ORGANIZATION_BLOCK MAIN:OB1
TITLE= Ciclo elettropneumatico A+/B+/A-/B- (ciclo quadro)
// Simulatore: 05
// Versione: 1.0
// Data: 28/02/2002
//------------     DESCRIZIONE  ---------------------
// L'esempio utilizza due cilindri (A e B) a doppio effetto e due
// elettrovalvole 5/2 bistabili (1V1 e 2V1).
// Una valvola 3/2 monostabile 0V permette la distribuzione dell'aria al
// circuito.
// Sulla mandata di ciascun cilindro sono preseti degli strozzatori
// unidirezionali che permettono di regolare separatamente la velocità
// delle singole corse dei pistoni.
// Un circuito di sicurezza, esterno al PLC, provvede (quando disattivato)
// a far rientrare lo stelo dei cilindri nella posizione di riposo
// (A0 B0)indipendentemente dalle uscite del PLC che vengono invece
// disattivate mediante un contatto del circuito di sicurezza
// (simulato dal Pulsante SB5). L'intervento di detto circuito
// non toglie però l'erogazione dell'aria compressa al circuito.
// Il ciclo continuo inizia con la pressione del pulsante SB1 e potrà
// essere interrotto mediante il pulsante di Stop SB3.
// Il pulsante SB2 permette di effetuare un solo ciclo quando premuto.
// Agli ingressi del PLC vengono collegati:
// - il selettore SB6 per il comando dell'aria compressa;
// - il pulsante di arresto ciclo SB3;
// - il pulsante di avvio ciclo in semiautomatico SB2;
// - il pulsante di avvio ciclo automatico SB1;
// - i fine corsa magnetici a0, a1, b0, b1 per il controllo
//   della posizione dei pistoni dei cilindri A e B;
// - il contatto di consenso del circuito di sicurezza (simulato dal
//   pulsante SB5).
//

BEGIN
NETWORK 1 // Controllo Distribuzione aria
//
LD I0.0 //SA
= Q0.0 //E_0Y1

NETWORK 2 // Controllo Merker fine ciclo
//
LD I1.0 //P_SB5
A I0.1 //P_SB3
= M0.2 //Fine Ciclo

NETWORK 3 // Controllo Merker Ciclo Automatico
//
LD I0.2 //P_SB1
O M0.1 //Ciclo ON
A M0.2 //Fine Ciclo
A I0.1 //P_SB3
= M0.1 //Ciclo ON

NETWORK 4 // Corsa A+
//
LD M0.1 //Ciclo ON
O I0.3 //P_SB2
A I0.6 //b0
A M0.2 //Fine Ciclo
= Q0.1 //E_1Y1

NETWORK 5 // Corsa A-
//
LD I0.7 //b1
A M0.2 //Fine Ciclo
= Q0.2 //E_1Y2

NETWORK 6 // Corsa B+
//
LD I0.5 //a1
A M0.2 //Fine ciclo
= Q0.3 //E_2Y1

NETWORK 7 // Corsa B-
//
LD I0.4 //a0
AN I0.6 //b0
A M0.2 //Fine ciclo
= Q0.4 //E_2Y2

NETWORK 8 // Segnalazione presenza Aria
//
LD Q0.0 //E_0Y1
= Q0.5 //HL1

NETWORK 9 // Segnalazione ciclo in funzione
//
LD M0.1 //Ciclo ON
= Q0.6 //HL2

END_ORGANIZATION_BLOCK

